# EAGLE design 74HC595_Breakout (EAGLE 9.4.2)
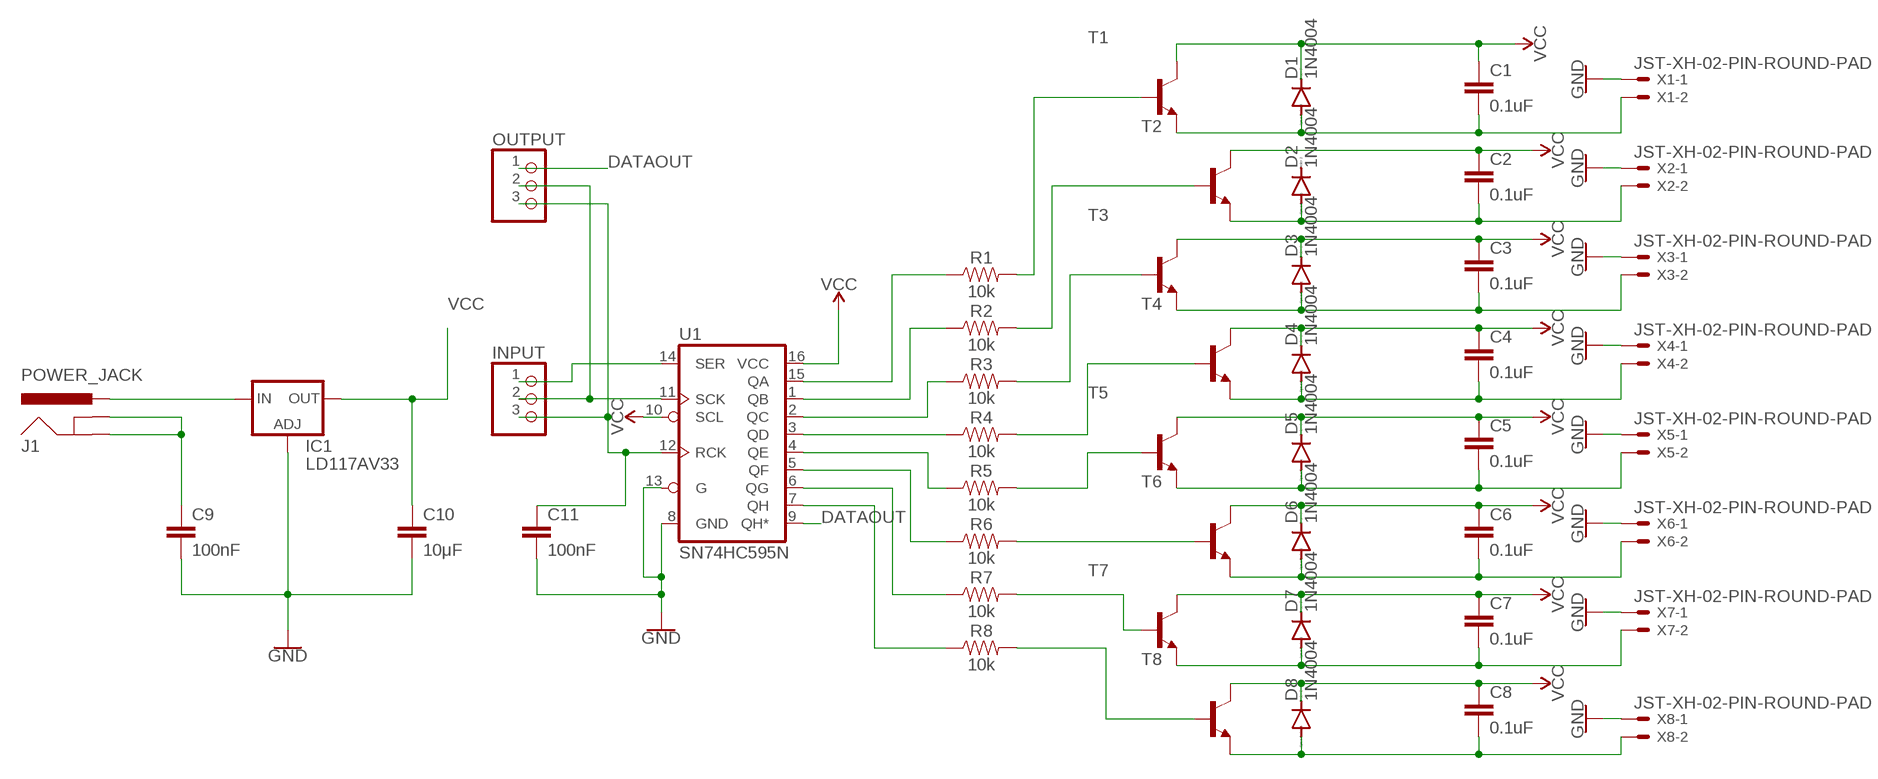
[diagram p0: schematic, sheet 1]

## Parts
C1  0.1uF  0.1UF-KIT-EZ-50V-20%  [CAP-PTH-SMALL-KIT]
C2  0.1uF  0.1UF-KIT-EZ-50V-20%  [CAP-PTH-SMALL-KIT]
C3  0.1uF  0.1UF-KIT-EZ-50V-20%  [CAP-PTH-SMALL-KIT]
C4  0.1uF  0.1UF-KIT-EZ-50V-20%  [CAP-PTH-SMALL-KIT]
C5  0.1uF  0.1UF-KIT-EZ-50V-20%  [CAP-PTH-SMALL-KIT]
C6  0.1uF  0.1UF-KIT-EZ-50V-20%  [CAP-PTH-SMALL-KIT]
C7  0.1uF  0.1UF-KIT-EZ-50V-20%  [CAP-PTH-SMALL-KIT]
C8  0.1uF  0.1UF-KIT-EZ-50V-20%  [CAP-PTH-SMALL-KIT]
C9  100nF  10NF-PTH-10MM-10000V-1-%  [CAP-PTH-10MM]
C10  10μF  10NF-PTH-10MM-10000V-1-%  [CAP-PTH-10MM]
C11  100nF  10NF-PTH-10MM-10000V-1-%  [CAP-PTH-10MM]
D1  1N4004  [DO41-10]
D2  1N4004  [DO41-10]
D3  1N4004  [DO41-10]
D4  1N4004  [DO41-10]
D5  1N4004  [DO41-10]
D6  1N4004  [DO41-10]
D7  1N4004  [DO41-10]
D8  1N4004  [DO41-10]
IC1  LD117AV33  [TO220L1]
INPUT  PINHD-1X3  [1X03]
J1  POWER_JACK  [POWER_JACK_PTH]
OUTPUT  PINHD-1X3  [1X03]
R1  10k  10KOHM-HORIZ-1/4W-1%  [AXIAL-0.3]
R2  10k  10KOHM-HORIZ-1/4W-1%  [AXIAL-0.3]
R3  10k  10KOHM-HORIZ-1/4W-1%  [AXIAL-0.3]
R4  10k  10KOHM-HORIZ-1/4W-1%  [AXIAL-0.3]
R5  10k  10KOHM-HORIZ-1/4W-1%  [AXIAL-0.3]
R6  10k  10KOHM-HORIZ-1/4W-1%  [AXIAL-0.3]
R7  10k  10KOHM-HORIZ-1/4W-1%  [AXIAL-0.3]
R8  10k  10KOHM-HORIZ-1/4W-1%  [AXIAL-0.3]
T1  2N3904-NPN-TO92-EBC  [TO92-EBC]
T2  2N3904-NPN-TO92-EBC  [TO92-EBC]
T3  2N3904-NPN-TO92-EBC  [TO92-EBC]
T4  2N3904-NPN-TO92-EBC  [TO92-EBC]
T5  2N3904-NPN-TO92-EBC  [TO92-EBC]
T6  2N3904-NPN-TO92-EBC  [TO92-EBC]
T7  2N3904-NPN-TO92-EBC  [TO92-EBC]
T8  2N3904-NPN-TO92-EBC  [TO92-EBC]
U1  SN74HC595N  74HC595N  [DIP16]
X1  JST-XH-02-PIN-ROUND-PAD  [JST-XH-02-PACKAGE-ROUND-PAD]
X2  JST-XH-02-PIN-ROUND-PAD  [JST-XH-02-PACKAGE-ROUND-PAD]
X3  JST-XH-02-PIN-ROUND-PAD  [JST-XH-02-PACKAGE-ROUND-PAD]
X4  JST-XH-02-PIN-ROUND-PAD  [JST-XH-02-PACKAGE-ROUND-PAD]
X5  JST-XH-02-PIN-ROUND-PAD  [JST-XH-02-PACKAGE-ROUND-PAD]
X6  JST-XH-02-PIN-ROUND-PAD  [JST-XH-02-PACKAGE-ROUND-PAD]
X7  JST-XH-02-PIN-ROUND-PAD  [JST-XH-02-PACKAGE-ROUND-PAD]
X8  JST-XH-02-PIN-ROUND-PAD  [JST-XH-02-PACKAGE-ROUND-PAD]

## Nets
DATAOUT: OUTPUT.1 U1.9(QH*)
GND: C9.2 C10.2 C11.2 IC1.1(ADJ) U1.8(GND) U1.13(G) X1.1 X2.1 X3.1 X4.1 X5.1 X6.1 X7.1 X8.1
N$2: R4.P$1 U1.3(QD)
N$3: R5.P$1 U1.4(QE)
N$4: R6.P$1 U1.5(QF)
N$5: R7.P$1 U1.6(QG)
N$6: R8.P$1 U1.7(QH)
N$7: R3.P$1 U1.2(QC)
N$8: R2.P$1 U1.1(QB)
N$9: R1.P$1 U1.15(QA)
N$10: R1.P$2 T1.B
N$11: R2.P$2 T2.B
N$12: R3.P$2 T3.B
N$13: R4.P$2 T4.B
N$14: R5.P$2 T5.B
N$15: R6.P$2 T6.B
N$16: R7.P$2 T7.B
N$17: R8.P$2 T8.B
N$18: C1.2 D1.A T1.E X1.2
N$19: C2.2 D2.A T2.E X2.2
N$20: C3.2 D3.A T3.E X3.2
N$21: C4.2 D4.A T4.E X4.2
N$22: C5.2 D5.A T5.E X5.2
N$23: C6.2 D6.A T6.E X6.2
N$24: C7.2 D7.A T7.E X7.2
N$25: C8.2 D8.A T8.E X8.2
N$26: IC1.3(IN) J1.PWR
N$27: C9.1 J1.GND J1.GNDBREAK
N$28: INPUT.1 U1.14(SER)
N$29: C11.1 INPUT.3 OUTPUT.3 U1.12(RCK)
N$30: INPUT.2 OUTPUT.2 U1.11(SCK)
VCC: C1.1 C2.1 C3.1 C4.1 C5.1 C6.1 C7.1 C8.1 C10.1 D1.C D3.C D4.C D5.C D6.C D7.C D8.C IC1.2(OUT) T1.C T2.C T3.C T4.C T5.C T6.C T7.C T8.C U1.10(SCL) U1.16(VCC)
Unconnected: D2.C

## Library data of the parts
C1-C8 = SparkFun-Capacitors:0.1UF: 0.1µF ceramic capacitors; PROD_ID: CAP-08370
C9-C11 = SparkFun-Capacitors:10NF: 0.01uF/10nF/10,000pF ceramic capacitors; PROD_ID: CAP-09321; VALUE: 10nF
D1-D8 = diode:1N4004: DIODE
IC1 = v-reg:LD117A?*: Low drop fixed and adjustable positive voltage regulators 1 A Source: http://www.st.com/stonline/products/literature/ds/7194/ld1117axx.pdf
INPUT OUTPUT = pinhead:PINHD-1X3: PIN HEADER
J1 = SparkFun-Connectors:POWER_JACK: Power Jack Connector This is the standard 5.5mm barrel jack for power. The PTH is the most common, proven, reliable, footprint. The Slot footprint only works if the mill layer is transmitted to the PCB fab house so be warned. Here are the connectors we sell at SparkFun: DC Barrel Power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; PROD_ID: CONN-08197
R1-R8 = SparkFun-Resistors:10KOHM: 10kΩ resistor; PROD_ID: RES-12183
T1-T8 = transistor-neu-to92:*-NPN-: NPN Transistror
U1 = SparkFun-IC-Logic:74*595: 8-Bit Shift Register (Serial to Parallel) Datasheet SparkFun Products SparkFun Shift Register Breakout - 74HC595 (BOB-10680); PROD_ID: IC-13123
X1-X8 = Rembrandt Electronics - JST XH Connectors v1-0:JST-XH-02-PIN: JST XH Connector 2 Pin

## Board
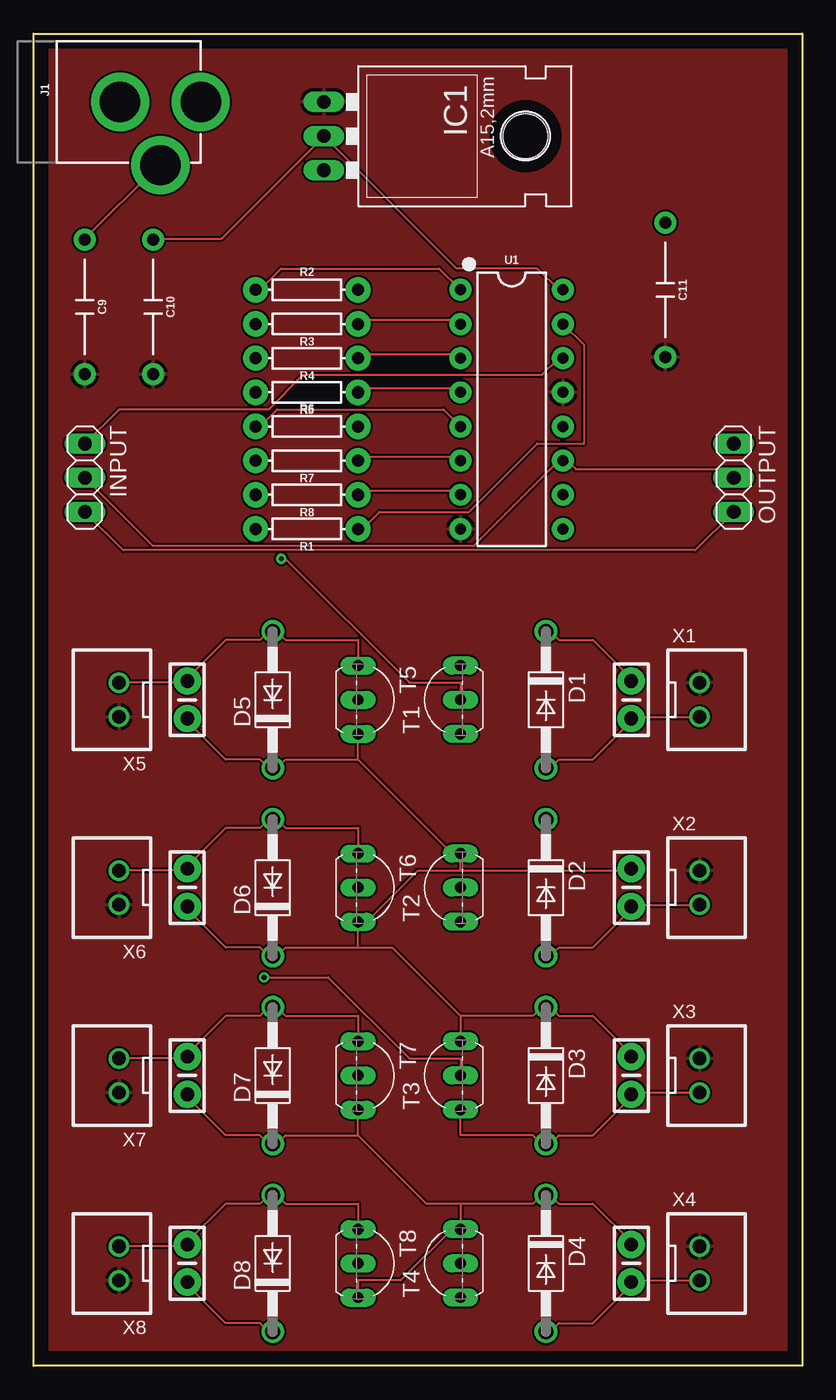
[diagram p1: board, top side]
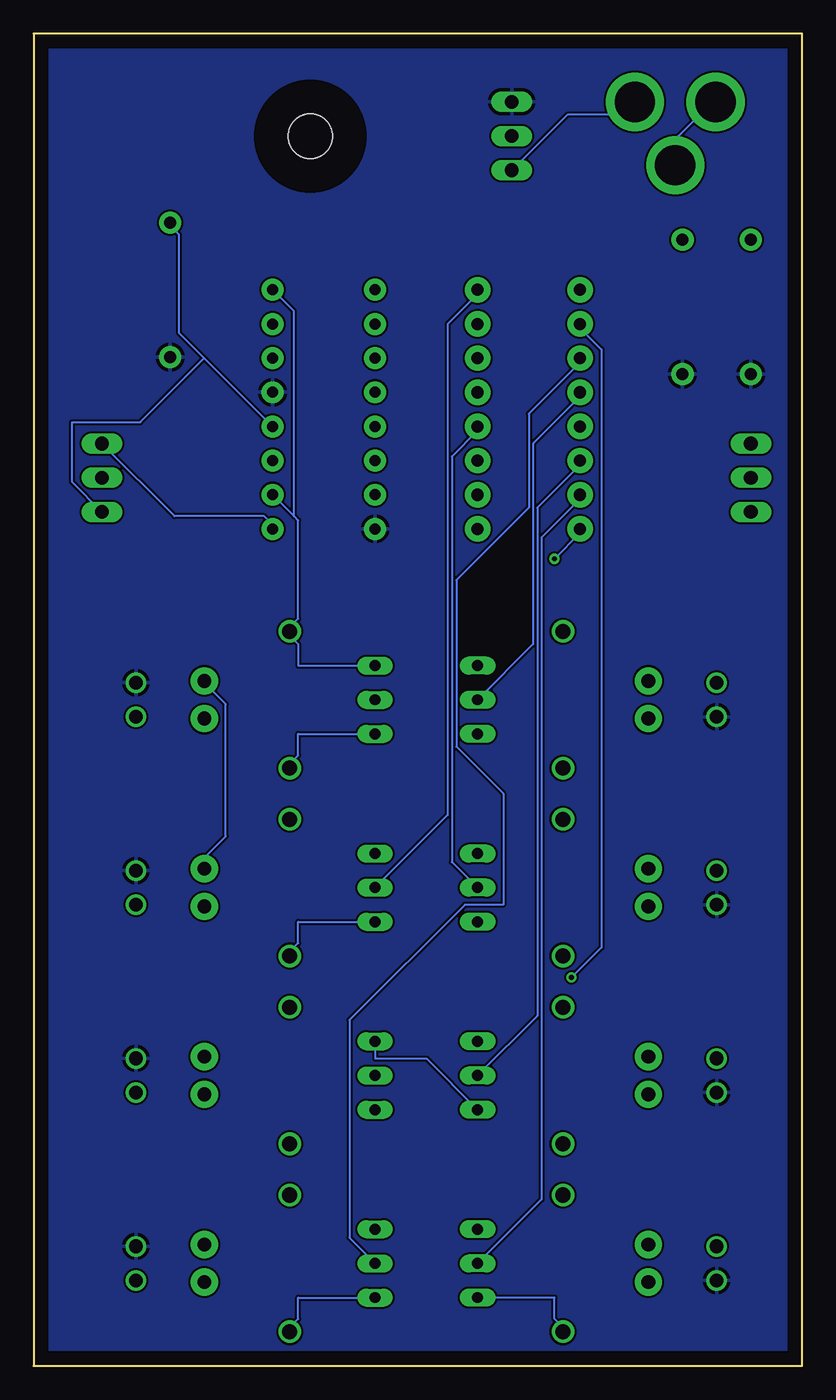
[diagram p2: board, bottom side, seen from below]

Size 57.15 x 99.06 mm. Coordinates in mm from the lower left corner, seen from the top.
Outline: 0,0 0,99.06 57.15,99.06 57.15,0 0,0
Copper layers (1*16): Top 0.035mm / dielectric 1.5mm / Bottom 0.035mm
Design rules "default": minimum track width 6mil, minimum drill 0.35mm, track to track 6mil, track to pad 6mil, pad to pad 6mil, via to via 6mil, smd to smd 6mil, copper to edge 40mil, drill to drill 6mil, minimum pad ring 10mil, minimum via ring 8mil, stop-mask expansion 4mil, vias tented up to drill 0mil, thermal gap 10mil

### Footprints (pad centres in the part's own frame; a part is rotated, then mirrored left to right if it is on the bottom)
CAP-PTH-SMALL-KIT = drill 1.016 pad 2.032: 1 -1.397,0; 2 1.397,0
CAP-PTH-10MM = drill 0.9 pad 1.651: 1 -5,0; 2 5,0
DO41-10 = drill 1.118: A 5.08,0; C -5.08,0
TO220L1 = drill 1.016 long: 1 -2.54,-3.81; 2 0,-3.81; 3 2.54,-3.81 | hole 3.302: 0,11.176
1X03 = drill 1.016 long: 1 -2.54,0; 2 0,0; 3 2.54,0
POWER_JACK_PTH = drill 2.997 pad 4.318: GND 0,7.7; GNDBREAK 4.7,10.7; PWR 0,13.7
AXIAL-0.3 = drill 0.9 pad 1.88: P$1 -3.81,0; P$2 3.81,0
TO92-EBC = drill 0.813 long: B 0,-1.27; C 2.54,-1.27; E -2.54,-1.27
DIP16 = drill 0.813 pad 1.626: 1 -8.89,-3.81; 2 -6.35,-3.81; 3 -3.81,-3.81; 4 -1.27,-3.81; 5 1.27,-3.81; 6 3.81,-3.81; 7 6.35,-3.81; 8 8.89,-3.81; 9 8.89,3.81; 10 6.35,3.81; 11 3.81,3.81; 12 1.27,3.81; 13 -1.27,3.81; 14 -3.81,3.81; 15 -6.35,3.81; 16 -8.89,3.81
JST-XH-02-PACKAGE-ROUND-PAD = drill 1.016: 1 -1.27,0; 2 1.27,0

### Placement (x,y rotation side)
C1  44.45,49.53 270 top
C2  44.45,35.56 270 top
C3  44.45,21.59 270 top
C4  44.45,7.62 270 top
C5  11.43,49.53 90 top
C6  11.43,35.56 90 top
C7  11.43,21.59 90 top
C8  11.43,7.62 90 top
C9  3.81,78.74 270 top
C10  8.89,78.74 270 top
C11  46.99,80.01 270 top
D1  38.1,49.53 270 top
D2  38.1,35.56 270 top
D3  38.1,21.59 270 top
D4  38.1,7.62 270 top
D5  17.78,49.53 90 top
D6  17.78,35.56 90 top
D7  17.78,21.59 90 top
D8  17.78,7.62 90 top
IC1  25.4,91.44 270 top
INPUT  3.81,66.04 270 top
J1  -1.27,93.98 270 top
OUTPUT  52.07,66.04 270 top
R1  20.32,62.23 180 top
R2  20.32,80.01 0 top
R3  20.32,77.47 180 top
R4  20.32,74.93 180 top
R5  20.32,72.39 180 top
R6  20.32,69.85 0 top
R7  20.32,67.31 180 top
R8  20.32,64.77 180 top
T1  30.48,49.53 90 top
T2  30.48,35.56 90 top
T3  30.48,21.59 90 top
T4  30.48,7.62 90 top
T5  25.4,49.53 270 top
T6  25.4,35.56 270 top
T7  25.4,21.59 270 top
T8  25.4,7.62 270 top
U1  35.56,71.12 270 top
X1  49.53,49.53 270 top
X2  49.53,35.56 270 top
X3  49.53,21.59 270 top
X4  49.53,7.62 270 top
X5  6.35,49.53 90 top
X6  6.35,35.56 90 top
X7  6.35,21.59 90 top
X8  6.35,7.62 90 top

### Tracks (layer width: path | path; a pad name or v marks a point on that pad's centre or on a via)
DATAOUT
  Bottom 0.152: OUTPUT.1 46.67,63.18 40.01,63.18 39.37,62.55 U1.9
GND
  pour Top (isolate 0): 0,0 0,99.06 57.15,99.06 57.15,0
  pour Bottom (isolate 0): 0,0 0,99.06 57.15,99.06 57.15,0
N$2
  Top 0.152: U1.3 31.43,75.25 24.45,75.25 R4.P$1
N$3
  Top 0.152: U1.4 31.43,72.71 24.45,72.71 R5.P$1
N$4
  Top 0.152: U1.5 30.48,71.12 18.1,71.12 16.83,69.85 R6.P$1
N$5
  Top 0.152: U1.6 31.43,67.63 24.45,67.63 R7.P$1
N$6
  Top 0.152: U1.7 31.43,65.09 24.45,65.09 R8.P$1
N$7
  Top 0.152: U1.2 31.43,77.79 24.45,77.79 R3.P$1
N$8
  Top 0.152: U1.1 30.16,81.6 18.41,81.6 16.83,80.01 R2.P$1
N$9
  Top 0.152: U1.15 40.96,75.88 40.96,68.58 37.47,68.58 32.38,63.5 25.72,63.5 24.45,62.23 R1.P$1
N$10  (via drill 0.35)
  Top 0.152: T1.B 31.75,50.8 27.94,50.8 18.73,60.01 v18.41,60.01
  Bottom 0.152: v18.41,60.01 16.51,61.91 R1.P$2
N$11
  Bottom 0.152: T2.B 26.35,40.96 26.35,77.47 24.13,79.69 R2.P$2
N$12  (via drill 0.35)
  Top 0.152: T3.B 31.75,22.86 27.94,22.86 21.91,28.89 v17.14,28.89
  Bottom 0.152: v17.14,28.89 14.92,31.11 14.92,75.56 16.51,77.15 R3.P$2
N$13
  Bottom 0.152: T4.B 33.66,9.53 33.66,25.72 25.08,34.29 22.23,34.29 22.23,42.55 25.72,46.04 25.72,58.42 20.32,63.82 20.32,70.8 16.51,74.61 R4.P$2
N$14
  Bottom 0.152: T5.B 20,53.66 20,68.58 16.51,72.07 R5.P$2
N$15
  Bottom 0.152: T6.B 26.04,37.47 26.04,67.63 24.13,69.53 R6.P$2
N$16
  Bottom 0.152: T7.B 19.68,26.04 19.68,63.82 16.51,66.99 R7.P$2
N$17
  Bottom 0.152: T8.B 19.37,12.38 19.37,61.59 16.51,64.45 R8.P$2
N$18
  Top 0.152: X1.2 44.45,48.26 C1.2 44.45,47.94 41.59,45.09 39.05,45.09 38.42,44.45 D1.A
  Bottom 0.152: T1.E 37.47,46.99 37.47,45.4 38.1,44.77 D1.A
N$19
  Top 0.152: X2.2 44.45,34.29 C2.2 44.45,33.97 41.59,31.11 39.05,31.11 38.42,30.48 D2.A
  Bottom 0.152: T2.E 37.47,33.02 37.47,31.43 38.1,30.8 D2.A
N$20
  Top 0.152: X3.2 44.45,20.32 C3.2 44.45,20 41.59,17.14 39.05,17.14 38.42,16.51 D3.A 37.78,16.51 37.15,17.14 31.75,17.14 T3.E
N$21
  Top 0.152: X4.2 44.45,6.35 C4.2 44.45,6.03 41.59,3.17 39.05,3.17 38.42,2.54 D4.A
  Bottom 0.152: T4.E 37.47,5.08 37.47,3.49 38.1,2.86 D4.A
N$22
  Top 0.152: X5.2 11.43,50.8 C5.2 11.43,51.12 14.29,53.98 16.83,53.98 17.46,54.61 D5.A 18.1,54.61 18.73,53.98 24.13,53.98 T5.E
N$23
  Top 0.152: X6.2 11.43,36.83 C6.2 11.43,37.15 14.29,40.01 16.83,40.01 17.46,40.64 D6.A 18.1,40.64 18.73,40.01 24.13,40.01 T6.E
N$24
  Top 0.152: X7.2 11.43,22.86 C7.2 11.43,23.18 14.29,26.04 16.83,26.04 17.46,26.67 D7.A 18.1,26.67 18.73,26.04 24.13,26.04 T7.E
N$25
  Top 0.152: X8.2 11.43,8.89 C8.2 11.43,9.21 14.29,12.06 16.83,12.06 17.46,12.7 D8.A 18.1,12.7 18.73,12.06 24.13,12.06 T8.E
N$26
  Bottom 0.152: IC1.3 17.46,93.03 12.7,93.03 12.7,93.98 J1.PWR
N$27
  Top 0.152: C9.1 3.81,83.82 9.21,89.22 J1.GNDBREAK
  Bottom 0.152: J1.GND 6.67,93.98 9.21,91.44 9.21,89.53 J1.GNDBREAK
N$28
  Top 0.152: INPUT.1 6.35,71.12 17.46,71.12 20,73.66 37.78,73.66 39.05,74.93 U1.14
N$29
  Top 0.152: INPUT.3 6.67,60.64 49.21,60.64 OUTPUT.3
  Bottom 0.152: 44.45,74.93 46.35,76.83 46.35,84.14 46.99,84.77 C11.1 | 44.45,74.93 U1.12 | 44.45,74.93 49.21,70.17 54.29,70.17 54.29,65.72 OUTPUT.3
N$30
  Top 0.152: INPUT.2 8.89,60.96 32.7,60.96 39.05,67.31 U1.11 39.69,67.31 40.32,66.67 51.44,66.67 OUTPUT.2
VCC
  Top 0.152: C10.1 8.89,83.82 13.97,83.82 IC1.2 31.43,81.6 37.47,81.6 39.05,80.01 U1.16 | D1.C 38.42,54.61 39.05,53.98 41.59,53.98 44.45,51.12 C1.1 | 24.13,17.14 T7.C | 24.13,17.14 18.73,17.14 18.1,16.51 D7.C 17.46,16.51 16.83,17.14 14.29,17.14 11.43,20 C7.1 | D8.C 17.46,2.54 16.83,3.17 14.29,3.17 11.43,6.03 C8.1 | 31.75,12.06 T4.C 31.11,10.16 27.3,6.35 24.13,6.35 T8.C | 31.75,12.06 37.15,12.06 37.78,12.7 D4.C 38.42,12.7 39.05,12.06 41.59,12.06 44.45,9.21 C4.1 | 24.13,17.14 29.21,12.06 31.75,12.06 | 31.75,26.04 T3.C | 31.75,26.04 37.15,26.04 37.78,26.67 D3.C 38.42,26.67 39.05,26.04 41.59,26.04 44.45,23.18 C3.1 | 24.13,45.09 T5.C | 24.13,45.09 18.73,45.09 18.1,44.45 D5.C 17.46,44.45 16.83,45.09 14.29,45.09 11.43,47.94 C5.1 | 24.13,31.11 T6.C 24.77,33.02 28.57,36.83 31.75,36.83 | 24.13,31.11 18.73,31.11 18.1,30.48 D6.C 17.46,30.48 16.83,31.11 14.29,31.11 11.43,33.97 C6.1 | 31.75,36.83 T2.C 31.11,38.1 24.13,45.09 | 31.75,36.83 44.45,36.83 C2.1 | 31.75,26.04 26.67,31.11 24.13,31.11
  Bottom 0.152: T1.C 37.47,52.07 37.47,53.66 38.1,54.29 D1.C 38.1,54.93 37.47,55.56 37.47,62.87 37.78,63.18 | 37.78,63.18 U1.10 | U1.16 37.78,78.42 37.78,63.18 | T8.C 18.41,5.08 18.41,3.49 17.78,2.86 D8.C | T7.C 27.94,22.86 31.75,22.86 T3.C | C2.1 44.45,37.78 42.86,39.37 42.86,49.21 44.45,50.8 C1.1

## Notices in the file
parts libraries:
SparkFun-IC-Logic: Licensing: Creative Commons ShareAlike 4.0 International - https://creativecommons.org/licenses/by-sa/4.0
